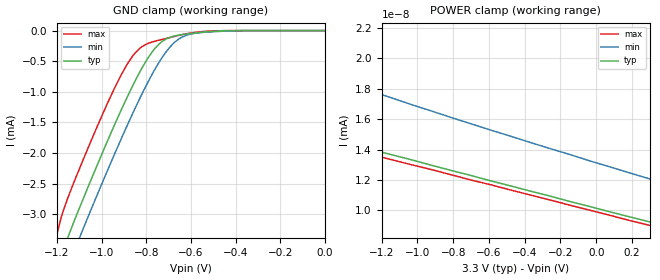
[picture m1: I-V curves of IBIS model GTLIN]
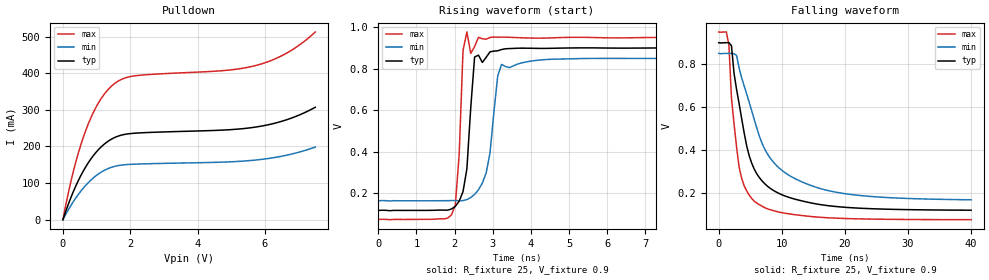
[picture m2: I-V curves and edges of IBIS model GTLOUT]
[IBIS Ver]   3.2
[Comment Char]   |_char
[File name]   gtl2034-.ibs
[File Rev]   0
[Date]   May 2, 2006 4:43:47 PM
[Source]
[Notes]
[Disclaimer]
* Specialty Logic Products for Philips Semiconductors. Tempe, AZ
* K.Williams
*  Property of Philips Semiconductors *
*  Unauthorized reproduction and/or distribution is strictly *
*  prohibited.  (C) Copyright 2005 Philips Semiconductors. *
*  All rights reserved. *
*  PLEASE BE AWARE THAT IN THE ABSENCE OF A SIGNED, WRITTEN AGREEMENT *
*  TO THE CONTRARY, PHILIPS SEMICONDUCTORS (COMPANY) IS PROVIDING THE *
*  SPICE MODELS "AS IS" AND WITHOUT ANY WARRANTY, EXPRESSED OR IMPLIED.  *
*  Further, COMPANY assumes no liability for: 1) the accuracy of the *
*  SPICE models provided to your company; 2) the proper functioning of *
*  these SPICE models in your design or for any resulting applications;  *
*  or 3) infringement of patents, copyrights or intellectual property *
*  rights resulting from your use of these SPICE models. *
*  COMPANY provides SPICE models as a service to our customers.  You and *
*  your company shall not distribute, convey, sell or give these models  *
*  to anyone else without receiving prior written permission from *
*  COMPANY. *
*  COMPANY reserves the right to make changes to its products or to *
*  discontinue any semiconductor product or service without notice and *
*  advises its customers to obtain the latest version of relevant *
*  information to verify, before placing orders, that the information *
*  being relied on is current. *
*  Please be aware that your receipt and subsequent use of the SPICE *
*  information provided shall serve as acceptance of the terms and *
*  conditions of this agreement.  If you do not accept these terms, *
*  you should return the SPICE model and any other accompanying *
*  information immediately. *
[Copyright]
[Component]   GTL2034
Si_location Pin
Timing_location Pin
[Manufacturer]   Philips Semiconductor
[Package]
R_pkg   34.6m   28.0m   44.6m
L_pkg   2.04n   1.36n   2.32n
C_pkg   0.37pf   0.30pf   0.44pf
[Pin] signal_name   model_name
1   NC   NC
2   Bo0   GTLOUT
3   Bo1   GTLOUT
4   VREF   POWER
5   Bo2   GTLOUT
6   Bo3   GTLOUT
7   GND   GND
8   GND   GND
9   Bi3   GTLIN
10   Bi2   GTLIN
11   GND   GND
12   Bi1   GTLIN
13   Bi0   GTLIN
14   VCC   POWER
| Models and submodels in the file (2): GTLIN (Input), GTLOUT (Open_drain)
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[Model]   GTLIN
Model_type Input
Vinh=0.65
Vinl=0.55
C_comp   4.5p   4.5p   4.5p
[Model Spec]
[Temperature Range] 27   85   -40
[Voltage Range]   3.3   3.0   3.6
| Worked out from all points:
|   GND clamp passes 1 mA (typ) near -0.87 V on its own axis
|   POWER clamp passes 1 mA (typ) near -9.27 V on its own axis
[GND Clamp]
-1.5V     -1.188A    -662.4mA   -2.047A
-1.2V     -3.93mA    -4.411mA   -3.324mA
-1.14V    -3.272mA   -3.764mA   -2.627mA
-1.08V    -2.726mA   -3.214mA   -2.087mA
-920mV    -1.359mA   -1.832mA   -777.7uA
-860mV    -893.5uA   -1.346mA   -410.3uA
-820mV    -614.8uA   -1.039mA   -263.8uA
-730mV    -180.1uA   -442.6uA   -145.3uA
-680mV    -93.21uA   -213.4uA   -100.6uA
-620mV    -56.36uA   -75.67uA   -52.02uA
-420mV    -1.852uA   -4.796uA   -323.8nA
0V        0A         -3.307fA   0A
[POWER Clamp]
-10.7V    21.08A     19.98A     22.42A
-3.92V    22.57pA    30.75pA    21.66pA
-3.81V    22.2pA     30.1pA     21.34pA
-3.59V    21.46pA    28.82pA    20.69pA
-3.37V    20.72pA    27.57pA    19.98pA
-2.81V    18.93pA    24.67pA    18.33pA
-2.7V     18.53pA    24.13pA    18.02pA
-2.14V    16.77pA    21.5pA     16.33pA
-1.59V    15.05pA    19.16pA    14.68pA
-1.03V    13.32pA    16.94pA    12.99pA
-370mV    11.27pA    14.47pA    11.01pA
300mV     9.237pA    12.07pA    9.01pA
[Model]   GTLOUT
Model_type Open_drain
Vref=0.9
Vmeas=0.6
Rref=25
C_comp   5.5p   5.5p   5.5p
[Model Spec]
[Temperature Range] 27   85   -40
[Voltage Range]   3.3   3.0   3.6
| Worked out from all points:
|   slope of the pulldown table from 0 to 0.495 V, typ, clamps not added: 4.37 ohm
|   falling waveform, R_fixture 25, V_fixture 0.9: 20-80 % time 3.85ns typ, 6.18ns min, 2.04ns max; typ from 0.9 V to 0.119 V
|   rising waveform, R_fixture 25, V_fixture 0.9: 20-80 % time 196ps typ, 269ps min, 135ps max; typ from 0.118 V to 0.9 V
[Pulldown]
0V        -5.986uA   -6.235uA   -6.613uA
300mV     74.39mA    47.83mA    127.9mA
450mV     105.1mA    67.92mA    179.2mA
680mV     144.5mA    93.97mA    243.7mA
1.06V     191.7mA    125.1mA    319.4mA
1.29V     210.7mA    137.4mA    349.7mA
1.52V     223.5mA    145.1mA    370.6mA
2.12V     236mA      151.5mA    392.5mA
4.77V     244.7mA    157.2mA    407mA
5.76V     253.3mA    163.1mA    421.6mA
6.67V     273.5mA    176.5mA    455.8mA
7.5V      306.9mA    198.3mA    512.5mA
[Falling Waveform]
R_fixture=25
V_fixture=0.9
V_fixture_min=0.85
V_fixture_max=0.95
0s        900mV      850mV      950mV
1.212ns   900mV      850mV      949.9mV
1.616ns   900.3mV    850.1mV    887.2mV
2.02ns    885.5mV    850mV      642.1mV
3.232ns   615.5mV    782mV      319.6mV
4.444ns   416.9mV    659.6mV    208.4mV
5.657ns   308.7mV    539.3mV    160mV
8.485ns   214.4mV    349.3mV    118.4mV
14.55ns   153.2mV    234.8mV    89.63mV
40ns      118.8mV    167.4mV    74.6mV
[Rising Waveform]
R_fixture=25
V_fixture=0.9
V_fixture_min=0.85
V_fixture_max=0.95
0s        117.6mV    164.2mV    74.25mV
1.919ns   124.5mV    165.1mV    96.22mV
2.02ns    137.5mV    165.3mV    143mV
2.121ns   162.2mV    164.3mV    385mV
2.222ns   208.5mV    165.1mV    888mV
2.323ns   317.8mV    170mV      977.3mV
2.525ns   856.6mV    195mV      907.1mV
2.828ns   855.3mV    298.2mV    942.6mV
3.232ns   892.7mV    821mV      952.5mV
10ns      900mV      850mV      949.9mV
[Ramp]
R_load=25
dV/dt_r   4.694E-1/1.710E-10   4.354E-1/2.577E-10   4.979E-1/1.086E-10
dV/dt_f   4.687E-1/3.841E-9   4.333E-1/6.281E-9   4.977E-1/2.010E-9
|[End   GTLOUT
